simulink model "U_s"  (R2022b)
settings: Solver=ode45  StartTime=0.0  StopTime=20  FixedStep=1  RelTol=1e-6  EnableMultiTasking=on
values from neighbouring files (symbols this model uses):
  Kp = 10    [para2Kp.m]

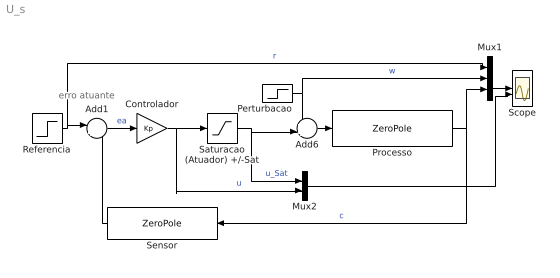
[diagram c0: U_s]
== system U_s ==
  note: erro atuante
  Add1 : Sum  Inputs=|+-
  Add6 : Sum  Inputs=++|
  Controlador : Gain  Gain=Kp
  Mux1 : Mux  Inputs=3
  Mux2 : Mux  Inputs=2
  Perturbacao : Step  Time=10  After=10  SampleTime=0
  Processo : ZeroPole  Zeros=[]  Poles=[-1 -2]
  Referencia : Step  Time=0  After=0  SampleTime=0
  Saturacao (Atuador) +/-Sat : Saturate  UpperLimit=10  LowerLimit=-10
  Scope : Scope  NumInputPorts=2
  Sensor : ZeroPole  Zeros=[]  Poles=[-10 ]  Gain=[10]
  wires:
  Mux1/1 -> Scope/1
  Processo/1 -> Mux1/3, Sensor/1  "c"
  Perturbacao/1 -> Add6/1, Mux1/2  "w"
  Add6/1 -> Processo/1
  Referencia/1 -> Add1/1, Mux1/1  "r"
  Mux2/1 -> Scope/2
  Saturacao (Atuador) +/-Sat/1 -> Mux2/1, Add6/2  "u_Sat"
  Add1/1 -> Controlador/1  "ea"
  Controlador/1 -> Mux2/2, Saturacao (Atuador) +/-Sat/1  "u"
  Sensor/1 -> Add1/2
